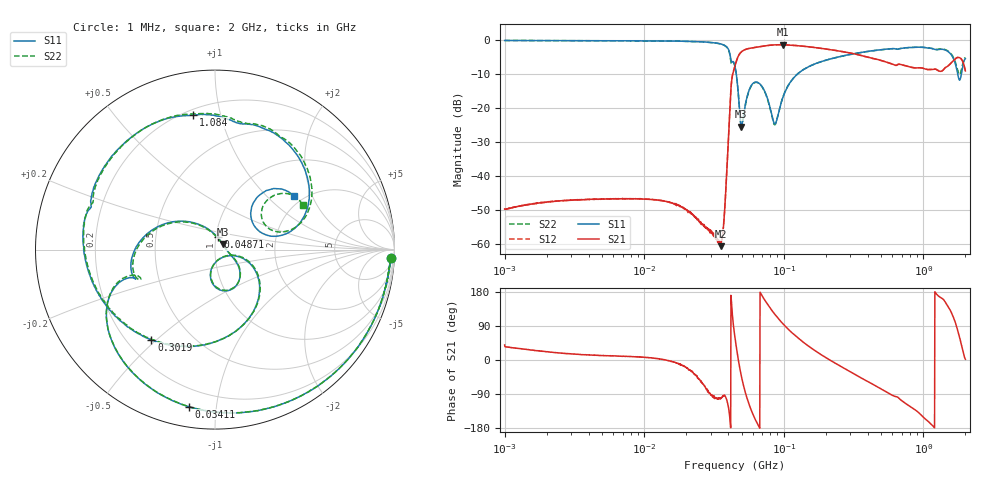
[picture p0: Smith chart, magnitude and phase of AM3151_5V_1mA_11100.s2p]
! Date/Time: Fri Jun 26 11:03:26 2020
! Network Analyzer:  Rev:
! Sweep from 1000000.0 to 2000000000.0, 1601 Points ! Power Supply: 0 V, 0 A
# HZ S DB R 50
!freq MagS11 AngS11 MagS21 AngS21 MagS12 AngS12 MagS22 AngS22
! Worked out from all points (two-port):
!   1601 points, 1 MHz to 2 GHz, reference 50 ohm
!   highest |S21| = -1.41 dB at 97.93 MHz (marker M1); lowest = -60.7 dB at 35.27 MHz (marker M2)
!   |S21| within 3 dB of the highest: 47.74 MHz to 345 MHz (297.3 MHz wide, 151 % of centre)
!   lowest |S11| = -25.5 dB at 49.65 MHz (marker M3), VSWR 1.11, Z = 54.5 + j3.31 ohm
!   |S11| at or under -10 dB: 45.66 MHz to 125.7 MHz (80.05 MHz wide, 93.4 % of centre); 1.761 GHz to 1.872 GHz (110.6 MHz wide, 6.09 % of centre)
!   |S22| runs from -25.8 to -0.2 dB; largest |S21 - S12| = 0.0092
!   S11 on the Smith chart (normalised r, x): 1 MHz: 16, -38; 34.11 MHz: 0.10, -0.84; 48.71 MHz: 1.02, +0.14; 301.9 MHz: 0.30, -0.48; 1.084 GHz: 0.23, +0.82; 2 GHz: 1.77, +1.48
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1000000  -0.16 -2.6  -49.73 39.7  -49.85 34.9  -0.17 -2.6
3555161  -0.22 -8.4  -46.98 14.2  -46.99 14.2  -0.22 -8.3
1.263916e7  -0.30 -29.5  -47.14 3.2  -47.17 3.2  -0.31 -29.4
2.310668e7  -0.47 -57.3  -52.20 -37.8  -51.99 -38.1  -0.47 -57.3
3.411262e7  -1.04 -99.4  -59.56 -99.9  -59.65 -102.0  -1.05 -99.8
3.526606e7  -1.16 -105.8  -60.67 -99.7  -59.96 -102.3  -1.19 -106.2
3.751269e7  -1.57 -120.7  -51.42 -93.8  -51.39 -93.3  -1.60 -121.4
4.204303e7  -6.32 -161.1  -13.22 159.8  -13.21 159.7  -6.88 -161.1
4.493426e7  -8.22 166.8  -7.29 53.1  -7.29 53.1  -8.27 168.0
4.871365e7  -23.10 77.9  -3.88 -27.0  -3.89 -27.1  -23.05 81.9
4.964819e7  -25.48 34.8  -3.53 -42.2  -3.53 -42.2  -25.80 40.0
5.51179e7  -16.07 -34.8  -2.60 -106.2  -2.60 -106.1  -16.27 -32.9
6.570964e7  -12.59 -78.1  -2.07 -172.9  -2.06 -173.0  -12.67 -77.4
8.573638e7  -24.62 -65.6  -1.46 121.9  -1.46 121.8  -24.91 -63.4
9.793384e7  -17.20 -16.7  -1.41 96.7  -1.42 96.7  -17.16 -15.1
1.589914e8  -7.41 -63.5  -2.13 30.4  -2.13 30.3  -7.42 -63.1
3.019241e8  -4.21 -125.1  -3.86 -32.0  -3.91 -31.9  -4.26 -125.7
5.652395e8  -2.64 175.3  -6.76 -88.2  -6.73 -88.1  -2.65 173.6
1.083636e9  -2.39 99.3  -8.72 -162.0  -8.71 -162.3  -2.35 96.8
1.511136e9  -3.49 41.4  -7.57 140.0  -7.53 139.1  -3.34 40.5
1.726123e9  -8.32 12.1  -5.28 89.5  -5.33 89.1  -7.62 14.4
2e9  -5.51 34.4  -9.13 1.8  -9.26 0.9  -5.23 26.8
